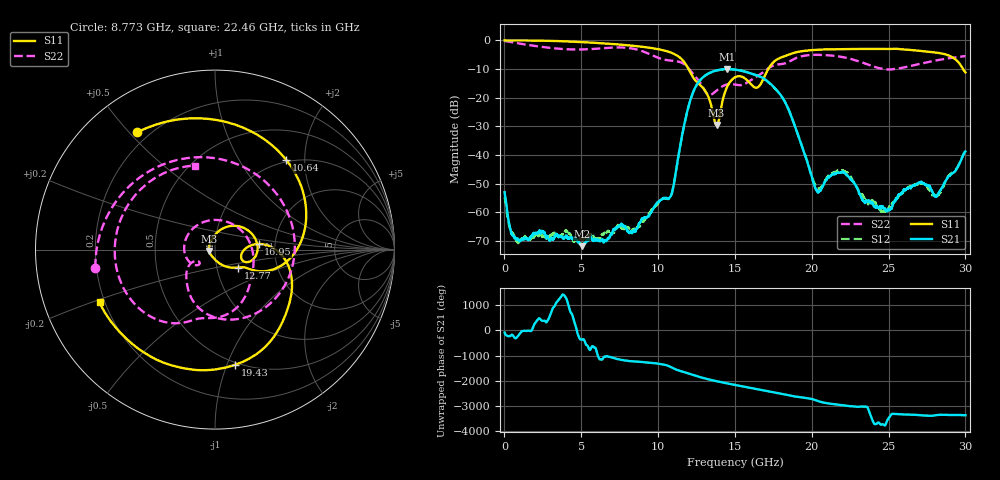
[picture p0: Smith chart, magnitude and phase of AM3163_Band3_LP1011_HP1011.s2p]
!Agilent Technologies,E8364B,MY43040894,A.07.50.67
!Agilent E8364B: A.07.50.67
!Date: Thursday, August 20, 2020 11:08:24
!Correction: S11(Full 2 Port(1,2))
!S21(Full 2 Port(1,2))
!S12(Full 2 Port(1,2))
!S22(Full 2 Port(1,2))
!S2P File: Measurements: S11, S21, S12, S22:
# Hz S  dB  R 50
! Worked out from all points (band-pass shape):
!   3201 points, 10 MHz to 30 GHz, reference 50 ohm
!   highest |S21| = -10.00 dB at 14.5 GHz (marker M1); lowest = -71.8 dB at 5.052 GHz (marker M2)
!   |S21| within 3 dB of the highest: 12.89 GHz to 16.78 GHz (3.889 GHz wide, 26.2 % of centre)
!   lowest |S11| = -29.5 dB at 13.81 GHz (marker M3), VSWR 1.07, Z = 46.8 - j0.719 ohm
!   |S11| at or under -10 dB: 11.98 GHz to 17.17 GHz (5.191 GHz wide, 35.6 % of centre); 29.84 GHz to end of sweep
!   |S22| runs from -19.1 to -0.2 dB; largest |S21 - S12| = 0.0067
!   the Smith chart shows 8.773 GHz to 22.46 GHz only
!   S11 on the Smith chart (normalised r, x): 8.773 GHz: 0.16, +0.53; 10.64 GHz: 0.97, +1.63; 12.77 GHz: 1.27, -0.26; 16.95 GHz: 1.64, +0.11; 19.43 GHz: 0.48, -1.07; 22.46 GHz: 0.18, -0.21
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1e7  -0.04 -2.0  -52.91 -94.7  -54.57 -71.3  -0.24 -5.8
1.143997e9  -0.04 -30.8  -69.35 -41.6  -69.53 15.3  -1.26 -83.6
2.512291e9  -0.14 -67.6  -66.60 7.5  -68.03 142.9  -2.35 -165.4
5.014581e9  -0.61 -132.5  -71.41 -17.1  -69.09 153.6  -3.18 62.8
5.052069e9  -0.62 -133.5  -71.75 -16.9  -69.37 -100.6  -3.17 60.8
6.279784e9  -1.00 -165.4  -69.88 -76.3  -68.18 53.1  -2.80 -7.9
7.413781e9  -1.43 164.2  -64.92 -67.8  -64.76 -53.0  -2.48 -76.6
8.772703e9  -2.11 123.5  -63.71 -167.3  -64.82 -166.4  -3.42 -171.4
1.000979e10  -3.08 79.0  -56.25 118.5  -56.72 119.1  -6.09 79.1
1.063771e10  -3.90 51.6  -55.20 37.3  -55.29 34.9  -6.95 15.6
1.153741e10  -6.57 2.8  -33.72 173.1  -33.95 173.0  -7.80 -71.7
1.277449e10  -15.72 -37.6  -13.62 -60.4  -13.69 -59.4  -15.05 -147.4
1.38054e10  -29.46 -166.8  -10.48 145.4  -10.52 145.7  -17.46 -139.3
1.449892e10  -16.14 57.2  -10.00 57.6  -10.10 58.4  -15.37 -175.5
1.5005e10  -12.87 20.4  -10.19 -2.2  -10.19 -1.0  -15.42 133.9
1.695435e10  -12.24 7.4  -13.57 135.9  -13.69 136.2  -10.66 -51.6
1.942852e10  -3.72 -80.1  -37.94 -140.2  -37.71 -139.0  -5.45 -141.7
2.000958e10  -3.39 -96.8  -47.65 161.4  -47.25 163.1  -5.09 -163.3
2.245564e10  -3.01 -155.4  -47.88 -118.3  -47.11 -116.0  -6.36 103.6
2.500479e10  -3.01 145.3  -58.97 124.3  -58.32 109.0  -10.17 -37.7
2.73665e10  -3.85 79.4  -50.25 -130.5  -49.95 -129.9  -7.81 -157.2
3e10  -11.17 -22.5  -38.77 -118.2  -38.49 -118.8  -5.48 113.0
